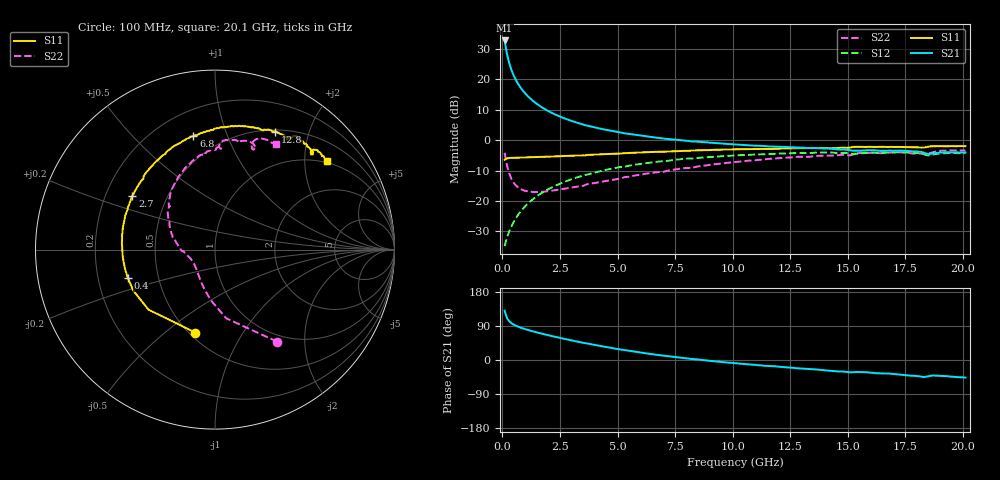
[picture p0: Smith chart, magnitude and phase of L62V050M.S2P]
!  Infineon Technologies AG
! BFR380L3 , PF131585-7, No.6, Th 09.10.01, soldered on pcb-board, measured with PP GSG850
!  Vce=2.0 V,  Ic=50.0 mA
! Common Emitter S-Parameters:  15. November 2001
#  GHz  S  MA  R  50
! f  S11  S21  S12  S22
! GHz  Mag  Ang  Mag  Ang  Mag  Ang  Mag  Ang
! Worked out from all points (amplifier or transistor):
!   201 points, 100 MHz to 20.1 GHz, reference 50 ohm
!   highest |S21| = 32.8 dB at 100 MHz (marker M1)
!   |S21| within 3 dB of that: start of sweep to 169.1 MHz
!   unconditionally stable (mu >= 1): 849.5 MHz to 4.312 GHz; 18.39617 GHz to 18.42132 GHz
!   at 3.4 GHz: K = 1.02, MAG = 7.9 dB, |S12| = -11.9 dB
!   at 10.1 GHz: K = 0.96, MSG = 1.8 dB, |S12| = -5.0 dB
!   at 20.1 GHz: K = 0.99, MSG = 0.1 dB, |S12| = -4.2 dB
!   S11 on the Smith chart (normalised r, x): 100 MHz: 0.54, -0.64; 400 MHz: 0.33, -0.14; 2.7 GHz: 0.31, +0.27; 6.8 GHz: 0.35, +0.76; 12.8 GHz: 0.52, +1.50; 20.1 GHz: 0.95, +2.57
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0.1  0.4757 -103.3  43.68 130.0  0.01801 59.4  0.6188 -56.0
0.2  0.4992 -138.0  26.5 110.9  0.02491 57.7  0.3879 -80.7
0.3  0.5093 -153.3  18.55 102.3  0.03142 61.0  0.2838 -94.6
0.4  0.5106 -162.1  14.18 97.0  0.03852 63.7  0.2294 -104.7
0.5  0.5129 -168.0  11.45 93.2  0.04541 66.0  0.1979 -112.7
0.6  0.5137 -172.6  9.59 90.2  0.05274 67.5  0.1783 -119.3
0.7  0.5158 -176.1  8.273 87.6  0.06007 68.5  0.1652 -124.9
0.8  0.516 -179.2  7.257 85.3  0.06747 69.2  0.1562 -129.6
0.9  0.518 178.2  6.468 83.3  0.07485 69.6  0.15 -133.8
1.1  0.5208 173.6  5.327 79.5  0.0897 69.6  0.144 -140.7
1.4  0.5267 167.6  4.218 74.4  0.112 69.0  0.1402 -148.4
1.7  0.5301 162.4  3.5 69.7  0.1343 67.8  0.1416 -154.5
2.1  0.5355 155.8  2.868 63.9  0.1635 65.6  0.1468 -160.6
2.7  0.5499 146.8  2.279 55.7  0.2061 61.8  0.159 -168.8
3.5  0.5614 136.1  1.809 45.6  0.2613 56.1  0.1768 -177.0
5.1  0.6 117.5  1.339 28.0  0.3607 44.1  0.2319 165.8
6.8  0.6438 100.8  1.086 13.0  0.4463 32.0  0.2984 147.8
10.1  0.7052 77.0  0.8493 -8.4  0.5592 10.2  0.4367 120.3
12.8  0.7376 63.1  0.7567 -21.8  0.6139 -6.2  0.5312 99.5
13.5  0.7402 59.8  0.742 -24.5  0.6188 -10.1  0.5422 95.2
16.8  0.7735 47.5  0.6741 -35.8  0.623 -25.6  0.6259 75.6
20.1  0.7969 38.3  0.6302 -46.5  0.617 -39.0  0.6801 60.1
